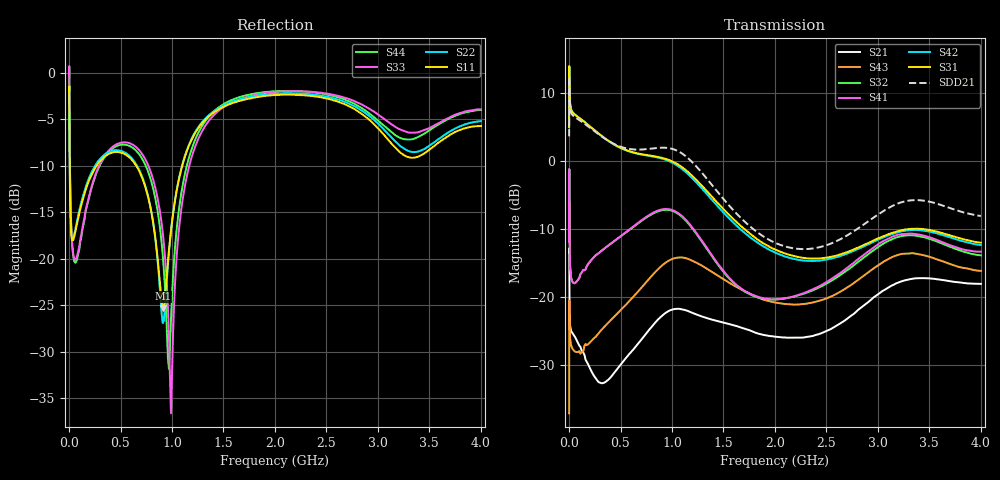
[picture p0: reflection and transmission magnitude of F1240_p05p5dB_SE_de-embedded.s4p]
! Integrated Device Technology
! Corporate Headquarters
! 6024 Silver Creek Valley Road
! San Jose, CA 95138  USA
! Phone:  1-408-284-8200
! Toll Free:  1-800-223-1366
! Webpage:  http://www.idt.com/
! Timing and RF Division
! 515 Groton Road, Suite 102
! Westford, MA 01886-6024
! Device:  F1240
! Description: Dual Intermediate Frequency Digital Variable Gain Amplifier
! Frequency:  10.0 -  500.00 MHz
! Package:  5x5 mm QFN Plastic Package: 32 pin
! Ports:  8 RF, 20 DC
!  Pin  1  = GA3 / Data  Pin 17  = RF OUT_B+
!  Pin  2  = GA4 / CLK  Pin 18  = RF OUT_B-
!  Pin  3  = GA5  Pin 19  = STBY_B
!  Pin  4  = VMODE  Pin 20  = Ground
!  Pin  5  = No Connect  Pin 21  = Ground
!  Pin  6  = GB5  Pin 22  = STB_A
!  Pin  7  = GB4  Pin 23  = RF OUT_A-  = Port 4
!  Pin  8  = GB3  Pin 24  = RF OUT_A+  = Port 3
!  Pin  9  = GB2  Pin 25  = GA0
!  Pin 10  = GB1  Pin 26  = ISET_A
!  Pin 11  = RF IN_B+  Pin 27  = VCC
!  Pin 12  = RF IN_B-  Pin 28  = Ground
!  Pin 13  = Ground  Pin 29  = RF IN_A-  = Port 2
!  Pin 14  = VCC  Pin 30  = RF IN_A+  = Port 1
!  Pin 15  = ISET_B  Pin 31  = GA1
!  Pin 16  = GB0  Pin 32  = GA2 / CSb
! Gain  = +19.5 dB
! State  = 1
! Voltage  = +5.00 V
! Current  = 85.292 mA (one channel only)
! Temperture  =  +25 C
! Test Date  =  2017-10-18
! Board  =  EB4031
! Data:  The device was measured on a custom evaluation board which has
!  individual transmission lines to the RF pins.  Data was collected
!  using a calibrated network analyzer.  The evaluation board was
!  de-embedded using Automatic Fixture Removal.
!  The reference plane is the edge of the package pin.
!  Only Channel A was measured.
!  This data is in single-ended operation.  If your needs are balanced
!  or differential S-parameters then this file needs to be used a
!  linear simulator.
! File Date:  2017-11-10  MJV
! Note:
!  Integrated Device Technology supplies this data as a sample of measured
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# Hz S dB R 100
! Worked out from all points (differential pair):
!   410 points, 500 kHz to 4 GHz, reference 100 ohm
!   strongest paths, dB at 500 kHz, 930 MHz, 1.96 GHz, 2.98 GHz, 4 GHz:
!     S31: 4.9, 0.3, -12.8, -11.6, -12.1
!     S42: 4.9, 0.2, -13.2, -11.8, -12.4
!     S41: -11.9, -7.1, -20.4, -12.5, -13.4
!     S32: -11.9, -7.2, -20.4, -12.9, -13.9
!     S43: -37.2, -15.1, -20.7, -15.6, -16.2
!     S21: -13.5, -22.5, -25.8, -19.9, -18.1
!   taken as a pair (ports 1,2 in; 3,4 out), SDD21 dB: 3.6, 1.9, -11.8, -8.1, -8.1
!   lowest |S11| = -25.3 dB at 910 MHz (marker M1), VSWR 1.11, Z = 90.4 - j3.71 ohm
!   |S11| at or under -10 dB: 6.47 MHz to 266.3 MHz (259.8 MHz wide, 191 % of centre); 652.5 MHz to 1.099 GHz (446.8 MHz wide, 51 % of centre)
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500000  -2.03 -5.5  -13.47 -5.7  -28.06 82.6  -44.96 78.9
        -13.48 -5.7  -2.03 -5.5  -44.99 78.1  -28.06 83.7
        4.95 -105.4  -11.92 -103.5  -0.45 1.3  -37.23 -72.4
        -11.91 -102.4  4.93 -104.3  -37.18 -72.7  -0.46 3.6
2500000  -3.35 -51.5  -16.52 -54.0  -16.78 31.8  -35.99 2.0
         -16.54 -54.0  -3.32 -51.4  -35.94 1.7  -16.79 32.1
         13.54 -176.2  -2.99 160.8  -0.77 -51.3  -20.62 -154.0
         -3.04 160.8  13.53 -175.9  -20.59 -154.0  -0.82 -50.9
4500000  -7.66 -68.7  -21.58 -46.2  -16.52 14.2  -38.70 -11.3
         -21.59 -46.2  -7.61 -68.8  -38.65 -11.5  -16.53 14.3
         11.06 165.6  -10.08 136.3  -4.87 -76.1  -23.30 174.7
         -10.14 136.3  11.06 165.8  -23.26 174.7  -4.94 -76.0
3e7  -18.02 -91.4  -25.27 -20.2  -17.02 -8.2  -41.03 2.7
     -25.29 -20.3  -17.83 -92.1  -41.05 3.1  -17.00 -8.1
     7.21 161.7  -17.73 131.7  -18.34 -129.0  -27.65 157.3
     -17.78 132.1  7.24 161.7  -27.56 157.4  -18.53 -129.6
1.9e8  -11.68 -130.3  -30.11 -48.8  -18.50 -48.6  -36.12 5.3
       -30.13 -48.2  -11.41 -131.4  -36.15 6.2  -18.52 -48.8
       5.21 111.6  -15.08 37.2  -13.42 -121.9  -27.13 96.9
       -15.13 37.2  5.20 111.0  -26.95 96.4  -13.57 -121.1
9.1e8  -25.34 -157.8  -22.92 -101.5  -18.32 164.1  -27.85 -145.6
       -22.73 -105.2  -26.90 -158.7  -27.98 -139.3  -18.65 163.0
       0.40 -72.8  -7.27 179.4  -17.20 137.8  -15.78 -84.6
       -7.14 176.2  0.28 -74.9  -15.33 -85.7  -19.64 143.1
4e9  -5.72 -142.0  -18.17 98.1  -23.02 -62.3  -23.95 -43.5
     -18.12 97.6  -5.19 -140.8  -24.75 -26.5  -24.63 -56.5
     -12.07 23.2  -13.93 -87.6  -3.92 -137.4  -17.24 72.6
     -13.39 -101.6  -12.42 29.3  -16.21 58.8  -3.98 -146.2
